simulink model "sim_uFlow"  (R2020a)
settings: Solver=ode15s  StartTime=0.0  StopTime=tsim  FixedStep=1  MaxStep=1  RelTol=1e-3
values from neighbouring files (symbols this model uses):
  dnom = [T0nom; TDnom; qDnom; Qnom]    [runTransformedMVs.m]
  Kc = 1/k*tau/(tauC+theta)    (= 0.000144927536232)    [runTransformedMVs.m]
  p = [V1;V2;rho;cp;A1;A2;tau01; tau02;transf]    [runTransformedMVs.m]
  T2nom = 30    [runTransformedMVs.m]
  tauI = min(tau,4*(tauC+theta))    [runTransformedMVs.m]
  Tnom = [T1nom;T2nom]    [runTransformedMVs.m]
  vbias = 0    [runTransformedMVs.m]
undefined symbols (not defined in the file or in its folder): CalcBlock, Tank

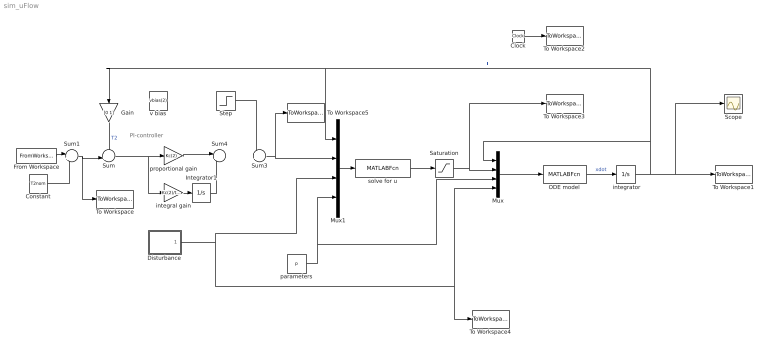
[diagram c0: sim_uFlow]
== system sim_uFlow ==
  note: PI-controller
  " integrator" : Integrator  InitialCondition=Tnom
  Clock : Clock
  Constant : Constant  Value=T2nom
  Disturbance : Subsystem
  From Workspace : FromWorkspace  VariableName=T2sp  OutputAfterFinalValue=Holding final value
  Gain : Gain  Gain=[0 1]  Multiplication=Matrix(K*u)
  Integrator1 : Integrator
  Mux : Mux
  Mux1 : Mux
  ODE model : MATLABFcn  MATLABFcn=Tank(u(1:2), u(3),u(4:12),u(13:16))  OutputDimensions=2
  Saturation : Saturate  UpperLimit=inf  LowerLimit=0
  Scope : Scope
  Step : Step  Time=10  Before=vbias(2)  After=vbias(2)-1  SampleTime=0
  Sum : Sum  Inputs=-+|
  Sum1 : Sum  Inputs=|++
  Sum3 : Sum  Inputs=++|
  Sum4 : Sum  Inputs=|++
  To Workspace : ToWorkspace  VariableName=Tsp  SampleTime=-1
  To Workspace1 : ToWorkspace  VariableName=T  SampleTime=-1
  To Workspace2 : ToWorkspace  VariableName=time  SampleTime=-1
  To Workspace3 : ToWorkspace  VariableName=u  SampleTime=-1
  To Workspace4 : ToWorkspace  VariableName=d  SampleTime=-1
  To Workspace5 : ToWorkspace  VariableName=v  SampleTime=-1
  integral gain : Gain  Gain=Kc(2)/tauI(2)  Multiplication=Matrix(K*u)
  parameters : Constant  Value=p
  proportional gain : Gain  Gain=Kc(2)  Multiplication=Matrix(K*u)
  solve for u : MATLABFcn  MATLABFcn=CalcBlock(u(1:2),u(3),u(4:7),u(8:16))  OutputDimensions=1
  v bias : Constant  Value=vbias(2)
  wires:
  " integrator"/1 -> To Workspace1/1, Scope/1, Gain/1, Mux1/1, Mux/1  "T"
  Mux/1 -> ODE model/1
  Clock/1 -> To Workspace2/1
  solve for u/1 -> Saturation/1
  Mux1/1 -> solve for u/1
  ODE model/1 -> " integrator"/1  "xdot"
  parameters/1 -> Mux/3, Mux1/4
  Saturation/1 -> Mux/2, To Workspace3/1
  Disturbance/1(d) -> Mux1/3, Mux/4, To Workspace4/1
  Sum1/1 -> Sum/2, To Workspace/1
  Gain/1 -> Sum/1  "T2"
  From Workspace/1 -> Sum1/1
  Constant/1 -> Sum1/2
  Sum3/1 -> To Workspace5/1, Mux1/2
  Sum/1 -> integral gain/1, proportional gain/1
  Integrator1/1 -> Sum4/2
  Step/1 -> Sum3/1
  integral gain/1 -> Integrator1/1
  proportional gain/1 -> Sum4/1
  Sum4/1 -> ?  "v1"

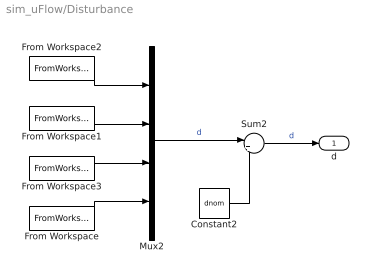
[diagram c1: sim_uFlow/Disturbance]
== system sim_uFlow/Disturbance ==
  Constant2 : Constant  Value=dnom
  From Workspace : FromWorkspace  VariableName=dist{4}  OutputAfterFinalValue=Setting to zero
  From Workspace1 : FromWorkspace  VariableName=dist{2}  OutputAfterFinalValue=Setting to zero
  From Workspace2 : FromWorkspace  VariableName=dist{1}  OutputAfterFinalValue=Setting to zero
  From Workspace3 : FromWorkspace  VariableName=dist{3}  OutputAfterFinalValue=Setting to zero
  Mux2 : Mux
  Sum2 : Sum  Inputs=|++
  d : Outport
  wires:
  From Workspace2/1 -> Mux2/1
  From Workspace/1 -> Mux2/4
  From Workspace3/1 -> Mux2/3
  Mux2/1 -> Sum2/1  "d"
  Constant2/1 -> Sum2/2
  From Workspace1/1 -> Mux2/2
  Sum2/1 -> d/1  "d"
